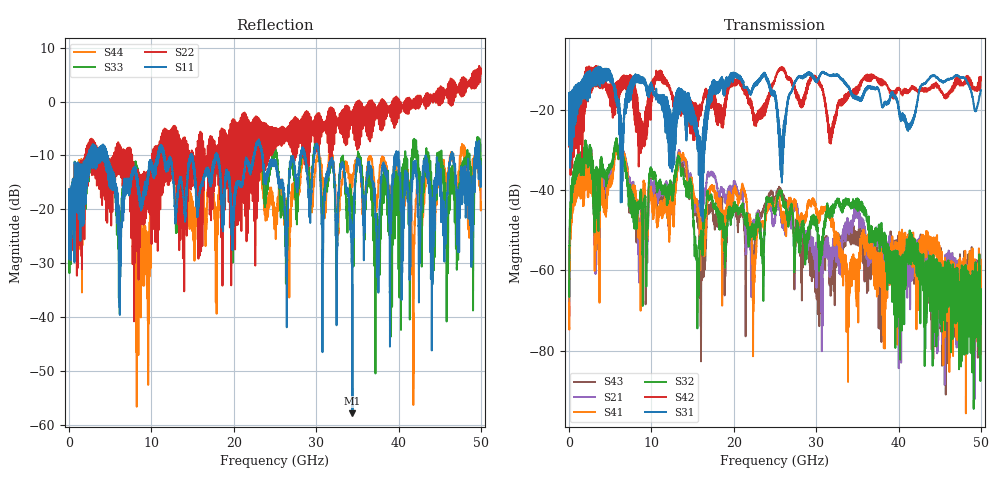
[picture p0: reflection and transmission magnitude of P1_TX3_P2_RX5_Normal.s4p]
!Keysight Technologies,N5225B,MY57041031,A.13.20.10
!Date: Friday, May 31, 2019 11:35:13
!Correction: S11(Full 4 Port(1,2,3,4))
!S12(Full 4 Port(1,2,3,4))
!S13(Full 4 Port(1,2,3,4))
!S14(Full 4 Port(1,2,3,4))
!S21(Full 4 Port(1,2,3,4))
!S22(Full 4 Port(1,2,3,4))
!S23(Full 4 Port(1,2,3,4))
!S24(Full 4 Port(1,2,3,4))
!S31(Full 4 Port(1,2,3,4))
!S32(Full 4 Port(1,2,3,4))
!S33(Full 4 Port(1,2,3,4))
!S34(Full 4 Port(1,2,3,4))
!S41(Full 4 Port(1,2,3,4))
!S42(Full 4 Port(1,2,3,4))
!S43(Full 4 Port(1,2,3,4))
!S44(Full 4 Port(1,2,3,4))
!S4P File: Measurements: <S11,S12,S13,S14>,
!<S21,S22,S23,S24>,
!<S31,S32,S33,S34>,
!<S41,S42,S43,S44>:
# Hz S  dB  R 50.0
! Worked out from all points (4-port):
!   5000 points, 10 MHz to 50 GHz, reference 50 ohm
!   strongest paths, dB at 10 MHz, 12.51 GHz, 25.01 GHz, 37.51 GHz, 50 GHz:
!     S31: -19.4, -27.1, -15.7, -14.5, -15.0
!     S42: -19.3, -17.3, -12.2, -12.7, -12.6
!     S32: -62.7, -41.7, -45.4, -51.7, -66.8
!     S41: -68.1, -42.7, -44.6, -59.9, -57.3
!     S21: -61.7, -40.0, -47.3, -51.2, -65.9
!     S43: -60.8, -43.2, -42.4, -57.0, -62.3
!   lowest |S11| = -57.9 dB at 34.41 GHz (marker M1), VSWR 1.00, Z = 49.9 + j0.11 ohm
!   |S11| at or under -10 dB: 4.66 GHz to 10.77 GHz (6.107 GHz wide, 79.2 % of centre); 23.49 GHz to 28.08 GHz (4.587 GHz wide, 17.8 % of centre); 30.37 GHz to 39.62 GHz (9.248 GHz wide, 26.4 % of centre)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
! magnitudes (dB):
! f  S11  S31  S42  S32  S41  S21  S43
! 10 MHz  -19.4  -19.4  -19.3  -62.7  -68.1  -61.7  -60.8
! 480 MHz  -21.7  -21.8  -24.1  -36.1  -40.3  -38.0  -38.3
! 2.07 GHz  -12.7  -12.5  -10.0  -29.2  -31.5  -30.4  -30.4
! 13.31 GHz  -16.1  -18.1  -18.2  -31.7  -31.5  -30.7  -31.8
! 15.61 GHz  -20.2  -29.9  -23.5  -57.0  -44.5  -42.9  -46.6
! 34.41 GHz  -57.9  -16.4  -16.1  -43.8  -60.5  -48.4  -49.2
! 50 GHz  -12.1  -15.0  -12.6  -66.8  -57.3  -65.9  -62.3
